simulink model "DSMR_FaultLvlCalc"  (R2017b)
settings: Solver=FixedStepDiscrete  StartTime=0.0  StopTime=10.0  FixedStep=0.02  RelTol=1e-3  EnableMultiTasking=on
undefined symbols (not defined in the file): bin2dec, BMS_DSMR_FaultLvlCalc, Delay, Delay1, DFES_Cls_DFC_638LinCommErr_C, DFES_Cls_DFC_AcDischgFobd_C, DFES_Cls_DFC_AChgFobd_C, DFES_Cls_DFC_AChgHVOffTmt_C, DFES_Cls_DFC_AChgHVOnTmt_C, DFES_Cls_DFC_AChgingErr_C, DFES_Cls_DFC_AChgLckTmt_C, DFES_Cls_DFC_AChgPileRdyTmt_C, DFES_Cls_DFC_AChgRdyPndiTmt_C, DFES_Cls_DFC_AChgRdyTmt_C, DFES_Cls_DFC_AChgS2ClsdTmt_C, DFES_Cls_DFC_AChgUnlckTmt_C, DFES_Cls_DFC_AChrgCnntErr_C, DFES_Cls_DFC_AChrgCurrMish_C, DFES_Cls_DFC_AChrgPortOvrTemp_C, DFES_Cls_DFC_AChrgVoltMish_C, DFES_Cls_DFC_AFEAdcRelatedErr_C, DFES_Cls_DFC_AFECellTempUpdErr_C, DFES_Cls_DFC_AFECellVoltLineOpen_C, DFES_Cls_DFC_AFECellVoltUpdErr_C, DFES_Cls_DFC_AFEComLost_C, DFES_Cls_DFC_AFEDiagModeExitErr_C, DFES_Cls_DFC_AFEGpioLineOpen_C, DFES_Cls_DFC_AFEOtherErr_C, DFES_Cls_DFC_AFEResetFlt_C, DFES_Cls_DFC_AFESampleErr_C, DFES_Cls_DFC_AFESplyFlt_C, DFES_Cls_DFC_AFETempHighFlt_C, DFES_Cls_DFC_APlusChk_C, DFES_Cls_DFC_BalCirOpenFlt_C, DFES_Cls_DFC_BalCirShortFlt_C, DFES_Cls_DFC_BalStuckMax_C, DFES_Cls_DFC_BalStuckMin_C, DFES_Cls_DFC_BalTempHighFlt_C, DFES_Cls_DFC_BattCurrMismatchErr_C, DFES_Cls_DFC_BattHVMsgTmt_C, DFES_Cls_DFC_BattSohChk_C, DFES_Cls_DFC_BattTAlrmMax_C, DFES_Cls_DFC_BattTAlrmMin_C, DFES_Cls_DFC_BattTCnstMax_C, DFES_Cls_DFC_BattTempVldMax_C, DFES_Cls_DFC_BattTempVldMin_C, DFES_Cls_DFC_BattTFaultMax_C, DFES_Cls_DFC_BattTFaultMin_C, DFES_Cls_DFC_BattTGradtMax_C, DFES_Cls_DFC_BattTHopMax_C, DFES_Cls_DFC_BattTWarnMax_C, DFES_Cls_DFC_BattTWarnMin_C, DFES_Cls_DFC_BattUNpl_C, DFES_Cls_DFC_BattVoltHiMax_C, DFES_Cls_DFC_BattVoltLoMin_C, DFES_Cls_DFC_BattVoltRngErr_C, DFES_Cls_DFC_BattVoltVld_C, DFES_Cls_DFC_BMSSplyPwrAbnToCAB_C, DFES_Cls_DFC_BMSSplyPwrAbnToLem_C, DFES_Cls_DFC_BoardTempTmt_C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
libraries: simulink x535
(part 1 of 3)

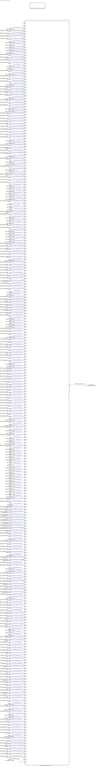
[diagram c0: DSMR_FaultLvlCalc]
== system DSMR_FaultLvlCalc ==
  DFC_CurrRngErr : Inport
  DFC_BattVoltRngErr : Inport  Port=2
  DFC_BattHVMsgTmt : Inport  Port=3
  DFC_BusHVMsgTmt : Inport  Port=4
  DFC_638LinCommErr : Inport  Port=5
  DFC_CellTempTmt : Inport  Port=6
  DFC_CellVoltTmt : Inport  Port=7
  DFC_InCanBusOff : Inport  Port=8
  DFC_VeCanBusOff : Inport  Port=9
  DFC_Msg2A3Tmt : Inport  Port=10
  DFC_RcMsg2A3Mis : Inport  Port=11
  DFC_ChkSumMsg2A3Err : Inport  Port=12
  DFC_RcMsg2A5Mis : Inport  Port=13
  DFC_RcMsg2A7Mis : Inport  Port=14
  DFC_CrashNpl : Inport  Port=15
  DFC_FuseNpl : Inport  Port=16
  DFC_Kl30cVoltLoErr : Inport  Port=17
  DFC_PosStuckMax : Inport  Port=18
  DFC_MPosStuckMin : Inport  Port=19
  DFC_MNegStuckMax : Inport  Port=20
  DFC_MNegStuckMin : Inport  Port=21
  DFC_PrStuckMin : Inport  Port=22
  DFC_DChrgPosStuckMax : Inport  Port=23
  DFC_DChrgPosStuckMin : Inport  Port=24
  DFC_DChrgNegStuckMax : Inport  Port=25
  DFC_DChrgNegStuckMin : Inport  Port=26
  DFC_HvPwrUpFail : Inport  Port=27
  DFC_DChrgPwrUpFail : Inport  Port=28
  DFC_BattTAlrmMax : Inport  Port=29
  DFC_BattTFaultMax : Inport  Port=30
  DFC_BattTAlrmMin : Inport  Port=31
  DFC_BattTFaultMin : Inport  Port=32
  DFC_BattTempVldMin : Inport  Port=33
  DFC_BattTCnstMax : Inport  Port=34
  DFC_BattTGradtMax : Inport  Port=35
  DFC_CellVoltAlrmMax : Inport  Port=36
  DFC_CellVoltFaultMax : Inport  Port=37
  DFC_CellVoltFusfMax : Inport  Port=38
  DFC_CellVoltAlrmMin : Inport  Port=39
  DFC_CellVoltFusfMin : Inport  Port=40
  DFC_CellVoltFaultMin : Inport  Port=41
  DFC_CellVoltVldMin : Inport  Port=42
  DFC_CellVoltNpl : Inport  Port=43
  DFC_Msg2E6Tmt : Inport  Port=44
  DFC_RcMsg2E6Mis : Inport  Port=45
  DFC_ChkSumMsg2E6Err : Inport  Port=46
  DFC_RcMsg2E1Mis : Inport  Port=47
  DFC_ChkSumMsg2E1Err : Inport  Port=48
  DFC_DcCanBusOff : Inport  Port=49
  DFC_DChrgTCnntMax : Inport  Port=50
  DFC_ChrgOCNpl : Inport  Port=51
  DFC_DisChOCNpl : Inport  Port=52
  DFC_BattVoltHiMax : Inport  Port=53
  DFC_BattVoltLoMin : Inport  Port=54
  DFC_ThmRnwy : Inport  Port=55
  DFC_AChrgPortOvrTemp : Inport  Port=56
  DFC_CurrOffsPlaus : Inport  Port=57
  DFC_CurrStukPlaus : Inport  Port=58
  DFC_CurrChrgPlaus : Inport  Port=59
  DFC_BattUNpl : Inport  Port=60
  DFC_BattVoltVld : Inport  Port=61
  DFC_PackUNpl : Inport  Port=62
  DFC_PackVoltVld : Inport  Port=63
  DFC_DChrgUNpl : Inport  Port=64
  DFC_DChrgVoltVld : Inport  Port=65
  DFC_BoardTempTmt : Inport  Port=66
  DFC_HvilMax : Inport  Port=67
  DFC_HvilMin : Inport  Port=68
  DFC_HvilSig : Inport  Port=69
  DFC_ChkSumMsg050Err : Inport  Port=70
  DFC_RcMsg050Mis : Inport  Port=71
  DFC_CrashHwNpl : Inport  Port=72
  DFC_IsoChkLv1 : Inport  Port=73
  DFC_IsoChkLv2 : Inport  Port=74
  DFC_InsResValdFault : Inport  Port=75
  DFC_Kl30OutRngErr : Inport  Port=76
  DFC_Kl30VoltLoErr : Inport  Port=77
  DFC_Kl30VoltHiErr : Inport  Port=78
  DFC_EepReadErr : Inport  Port=79
  DFC_BalStuckMax : Inport  Port=80
  DFC_BalStuckMin : Inport  Port=81
  DFC_CSCPwrSpyHiErr : Inport  Port=82
  DFC_CSCPwrSpyLoErr : Inport  Port=83
  DFC_CmcBordOTMax : Inport  Port=84
  DFC_BattTWarnMax : Inport  Port=85
  DFC_BattTWarnMin : Inport  Port=86
  DFC_BattTempVldMax : Inport  Port=87
  DFC_BattTHopMax : Inport  Port=88
  DFC_CellVoltRngHiErr : Inport  Port=89
  DFC_CellVoltRngLoErr : Inport  Port=90
  DFC_CellVoltWarnMax : Inport  Port=91
  DFC_CellVoltWarnMin : Inport  Port=92
  DFC_CellVoltVldMax : Inport  Port=93
  DFC_AChrgCurrMish : Inport  Port=94
  DFC_DChrgCurrMish : Inport  Port=95
  DFC_DChrgLowTempCurrMish : Inport  Port=96
  DFC_AChrgVoltMish : Inport  Port=97
  DFC_DChrgVoltMish : Inport  Port=98
  DFC_DChrgBattTMin : Inport  Port=99
  DFC_CC2Chk : Inport  Port=100
  DFC_APlusChk : Inport  Port=101
  DFC_DChrgMsgTmt : Inport  Port=102
  DFC_DChrgTNegElecMax : Inport  Port=103
  DFC_DChrgTNegElecMin : Inport  Port=104
  DFC_DChrgTNegElecSig : Inport  Port=105
  DFC_DChrgTPosElecMax : Inport  Port=106
  DFC_DChrgTPosElecMin : Inport  Port=107
  DFC_DChrgTPosElecSig : Inport  Port=108
  DFC_CcuSelfChkErr : Inport  Port=109
  DFC_ChrgOCMin : Inport  Port=110
  DFC_ChrgOCMax : Inport  Port=111
  DFC_DisChOCMin : Inport  Port=112
  DFC_DisChOCMax : Inport  Port=113
  DFC_SocRngLoMax : Inport  Port=114
  DFC_SocRngLoMin : Inport  Port=115
  DFC_SocRngHiMax : Inport  Port=116
  DFC_SocRngHiMin : Inport  Port=117
  DFC_InClntOverTmp : Inport  Port=118
  DFC_OutClntOverTmp : Inport  Port=119
  DFC_ClntDsTElecMax : Inport  Port=120
  DFC_ClntDsTElecMin : Inport  Port=121
  DFC_ClntDsTElecSig : Inport  Port=122
  DFC_ClntUsTElecMax : Inport  Port=123
  DFC_ClntUsTElecMin : Inport  Port=124
  DFC_ClntUsTElecSig : Inport  Port=125
  DFC_CoolPerfPlaus : Inport  Port=126
  DFC_HtgPerfPlaus : Inport  Port=127
  DFC_DChrgFobd : Inport  Port=128
  DFC_DChrgHvOnFail : Inport  Port=129
  DFC_AChgHVOnTmt : Inport  Port=130
  DFC_AChgHVOffTmt : Inport  Port=131
  DFC_AChgS2ClsdTmt : Inport  Port=132
  DFC_DChrgStakeErr : Inport  Port=133
  DFC_DChrgStkVoltErr : Inport  Port=134
  DFC_DChrgStkCurrErr : Inport  Port=135
  DFC_AChgPileRdyTmt : Inport  Port=136
  DFC_DChrgCHMTmt : Inport  Port=137
  DFC_DChrgCRMTmt : Inport  Port=138
  DFC_DChrgCMLTmt : Inport  Port=139
  DFC_DChrgCROTmt : Inport  Port=140
  DFC_DChrgCCSTmt : Inport  Port=141
  DFC_DChrgCSTTmt : Inport  Port=142
  DFC_DChrgCSDTmt : Inport  Port=143
  DFC_DChrgParaChk : Inport  Port=144
  DFC_DChrgCableChk : Inport  Port=145
  DFC_DChrgSLACTOut : Inport  Port=146
  DFC_DChrgCnntErr : Inport  Port=147
  DFC_DChrgLckErr : Inport  Port=148
  DFC_AChrgCnntErr : Inport  Port=149
  DFC_AChgLckTmt : Inport  Port=150
  DFC_AChgRdyPndiTmt : Inport  Port=151
  DFC_AChgRdyTmt : Inport  Port=152
  DFC_AChgingErr : Inport  Port=153
  DFC_AChgUnlckTmt : Inport  Port=154
  DFC_AChgFobd : Inport  Port=155
  DFC_SocValJmp : Inport  Port=156
  DFC_ChrgCmuLost : Inport  Port=157
  DFC_DisChrgCmuLost : Inport  Port=158
  DFC_Msg130Tmt : Inport  Port=159
  DFC_Msg2E1Tmt : Inport  Port=160
  DFC_Msg2EBTmt : Inport  Port=161
  DFC_MsgCABTmt : Inport  Port=162
  DFC_Msg0B5Tmt : Inport  Port=163
  DFC_ObcTmt : Inport  Port=164
  DFC_VcuTmt : Inport  Port=165
  DFC_Msg2A7Tmt : Inport  Port=166
  DFC_Msg2A5Tmt : Inport  Port=167
  DFC_Msg2ADTmt : Inport  Port=168
  DFC_Msg2BBTmt : Inport  Port=169
  DFC_Msg2DFTmt : Inport  Port=170
  DFC_Msg3AATmt : Inport  Port=171
  DFC_Msg050Tmt : Inport  Port=172
  DFC_Msg2F1Tmt : Inport  Port=173
  DFC_Msg195Tmt : Inport  Port=174
  DFC_Msg37FTmt : Inport  Port=175
  DFC_Msg28CTmt : Inport  Port=176
  DFC_Msg17DTmt : Inport  Port=177
  DFC_HwCurrElecSCG : Inport  Port=178
  DFC_HwCurrElecSCP : Inport  Port=179
  DFC_CABErr : Inport  Port=180
  DFC_BattCurrMismatchErr : Inport  Port=181
  GaCFM_AFEComLost_flg : Inport  Port=182
  GaCFM_AFECellVoltUpdErr_flg : Inport  Port=183
  GaCFM_AFECellTempUpdErr_flg : Inport  Port=184
  GaCFM_AFESampleErr_flg : Inport  Port=185
  GaCFM_AFECellVoltLineOpen_flg : Inport  Port=186
  GaCFM_AFEGpioLineOpen_flg : Inport  Port=187
  GaCFM_AFEAdcRelatedErr_flg : Inport  Port=188
  GaCFM_AFEDiagModeExitErr_flg : Inport  Port=189
  GaCFM_AFEOtherErr_flg : Inport  Port=190
  DFC_AcDischgFobd : Inport  Port=191
  DFC_BalCirOpenFlt : Inport  Port=192
  DFC_BalCirShortFlt : Inport  Port=193
  DFC_BalTempHighFlt : Inport  Port=194
  DFC_HVSmplComFlt : Inport  Port=195
  DFC_HVSmplSigErr : Inport  Port=196
  DFC_HVSmplSplyFlt : Inport  Port=197
  DFC_CABVoltOutOfRng : Inport  Port=198
  DFC_CABDevFlt : Inport  Port=199
  DFC_BMSSplyPwrAbnToLem : Inport  Port=200
  DFC_BMSSplyPwrAbnToCAB : Inport  Port=201
  DFC_NVMReadError : Inport  Port=202
  DFC_KL30Shutdown : Inport  Port=203
  DFC_MCUResetFlt : Inport  Port=204
  DFC_BattSohChk : Inport  Port=205
  DFC_CalCANBusOff : Inport  Port=206
  DFC_ThmRnwyWarn : Inport  Port=207
  DFC_PchgOvrCurrFlt : Inport  Port=208
  DFC_SBCSplyPwrOvrVolt : Inport  Port=209
  DFC_SBCSplyPwrUnderVolt : Inport  Port=210
  DFC_SBCSplyPwrOvrCurr : Inport  Port=211
  DFC_CrashChkHwFrqAbnorm : Inport  Port=212
  DFC_CrashChkHwDutyAbnorm : Inport  Port=213
  DFC_AFETempHighFlt : Inport  Port=214
  DFC_EVCCDevFlt : Inport  Port=215
  DFC_EVCCSplyPwrFlt : Inport  Port=216
  DFC_EVCCVehComFlt : Inport  Port=217
  DFC_EVCCPileComFlt : Inport  Port=218
  DFC_EVCCVehHwFlt : Inport  Port=219
  DFC_EVCCPileHwFlt : Inport  Port=220
  DFC_IsoS1SwStuckOpen : Inport  Port=221
  DFC_IsoS1SwStuckClsd : Inport  Port=222
  DFC_IsoS2SwStuckOpen : Inport  Port=223
  DFC_IsoS2SwStuckClsd : Inport  Port=224
  DFC_IsoS3SwStuckOpen : Inport  Port=225
  DFC_IsoS3SwStuckClsd : Inport  Port=226
  DFC_AFEResetFlt : Inport  Port=227
  DFC_AFESplyFlt : Inport  Port=228
  DFC_PreHeatErr : Inport  Port=229
  DFC_PreHeatVcuReqTmt : Inport  Port=230
  DFC_PreHeatObcStatusErr : Inport  Port=231
  DFC_PreHeatPtcErr : Inport  Port=232
  DFC_MPosRlyDrvScb : Inport  Port=233
  DFC_MPosRlyDrvScg : Inport  Port=234
  DFC_MPosRlyDrvOL : Inport  Port=235
  DFC_MposRlyDrvOvrCurr : Inport  Port=236
  DFC_MPosRlyDrvFault : Inport  Port=237
  DFC_MNegRlyDrvScb : Inport  Port=238
  DFC_MNegRlyDrvScg : Inport  Port=239
  DFC_MNegRlyDrvOL : Inport  Port=240
  DFC_MNegRlyDrvOvrCurr : Inport  Port=241
  DFC_MNegRlyDrvFault : Inport  Port=242
  DFC_DcPosRlyDrvScb : Inport  Port=243
  DFC_DcPosRlyDrvScg : Inport  Port=244
  DFC_DcPosRlyDrvOL : Inport  Port=245
  DFC_DChrgPosRlyDrvOvrCurr : Inport  Port=246
  DFC_DcPosRlyDrvFault : Inport  Port=247
  DFC_DcNegRlyDrvScb : Inport  Port=248
  DFC_DcNegRlyDrvScg : Inport  Port=249
  DFC_DcNegRlyDrvOL : Inport  Port=250
  DFC_DChrgNegRlyDrvOvrCurr : Inport  Port=251
  DFC_DcNegRlyDrvFault : Inport  Port=252
  DFC_PreRlyDrvScb : Inport  Port=253
  DFC_PreRlyDrvScg : Inport  Port=254
  DFC_PreRlyDrvOL : Inport  Port=255
  DFC_PrRlyDrvOvrCurr : Inport  Port=256
  DFC_CellTAlrmMax : Inport  Port=257
  DFC_CellTFaultMax : Inport  Port=258
  DFC_CellTAlrmMin : Inport  Port=259
  DFC_CellTFaultMin : Inport  Port=260
  DFC_CellTempVldMin : Inport  Port=261
  DFC_CellTCnstMax : Inport  Port=262
  DFC_CellTGradtMax : Inport  Port=263
  DFC_CellTWarnMax : Inport  Port=264
  DFC_CellTWarnMin : Inport  Port=265
  DFC_CellTempVldMax : Inport  Port=266
  DFC_CellTHopMax : Inport  Port=267
  DFC_TwoCurrSnsrFlt : Inport  Port=268
  DFC_ThmRnwyAlarm : Inport  Port=269
  DFC_ChkSumMsg2A5Err : Inport  Port=270
  DFC_ChkSumMsg2A7Err : Inport  Port=271
  DFC_DchrgIsoChkLv1 : Inport  Port=272
  DFC_DchrgIsoChkLv2 : Inport  Port=273
  DFC_HVOffIsoChkLv1 : Inport  Port=274
  DFC_HVOffIsoChkLv2 : Inport  Port=275
  DFC_PackCrntSaf : Inport  Port=276
  BMS_DSMR_FaultLvlCalc : Subsystem
  FaultLvlCoord_Clear_Function : Subsystem  TreatAsAtomicUnit=on
  DSMR_stFaultRank : Outport
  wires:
  DFC_CurrRngErr/1 -> BMS_DSMR_FaultLvlCalc/1(DFC_CurrRngErr)  "DFC_CurrRngErr"
  DFC_BattVoltRngErr/1 -> BMS_DSMR_FaultLvlCalc/2(DFC_BattVoltRngErr)  "DFC_BattVoltRngErr"
  DFC_BattHVMsgTmt/1 -> BMS_DSMR_FaultLvlCalc/3(DFC_BattHVMsgTmt)  "DFC_BattHVMsgTmt"
  DFC_BusHVMsgTmt/1 -> BMS_DSMR_FaultLvlCalc/4(DFC_BusHVMsgTmt)  "DFC_BusHVMsgTmt"
  DFC_638LinCommErr/1 -> BMS_DSMR_FaultLvlCalc/5(DFC_638LinCommErr)  "DFC_638LinCommErr"
  DFC_CellTempTmt/1 -> BMS_DSMR_FaultLvlCalc/6(DFC_CellTempTmt)  "DFC_CellTempTmt"
  DFC_CellVoltTmt/1 -> BMS_DSMR_FaultLvlCalc/7(DFC_CellVoltTmt)  "DFC_CellVoltTmt"
  DFC_InCanBusOff/1 -> BMS_DSMR_FaultLvlCalc/8(DFC_InCanBusOff)  "DFC_InCanBusOff"
  DFC_VeCanBusOff/1 -> BMS_DSMR_FaultLvlCalc/9(DFC_VeCanBusOff)  "DFC_VeCanBusOff"
  DFC_Msg2A3Tmt/1 -> BMS_DSMR_FaultLvlCalc/10(DFC_Msg2A3Tmt)  "DFC_Msg2A3Tmt"
  DFC_RcMsg2A3Mis/1 -> BMS_DSMR_FaultLvlCalc/11(DFC_RcMsg2A3Mis)  "DFC_RcMsg2A3Mis"
  DFC_ChkSumMsg2A3Err/1 -> BMS_DSMR_FaultLvlCalc/12(DFC_ChkSumMsg2A3Err)  "DFC_ChkSumMsg2A3Err"
  DFC_RcMsg2A5Mis/1 -> BMS_DSMR_FaultLvlCalc/13(DFC_RcMsg2A5Mis)  "DFC_RcMsg2A5Mis"
  DFC_RcMsg2A7Mis/1 -> BMS_DSMR_FaultLvlCalc/14(DFC_RcMsg2A7Mis)  "DFC_RcMsg2A7Mis"
  DFC_CrashNpl/1 -> BMS_DSMR_FaultLvlCalc/15(DFC_CrashNpl)  "DFC_CrashNpl"
  DFC_FuseNpl/1 -> BMS_DSMR_FaultLvlCalc/16(DFC_FuseNpl)  "DFC_FuseNpl"
  DFC_Kl30cVoltLoErr/1 -> BMS_DSMR_FaultLvlCalc/17(DFC_Kl30cVoltLoErr)  "DFC_Kl30cVoltLoErr"
  DFC_PosStuckMax/1 -> BMS_DSMR_FaultLvlCalc/18(DFC_PosStuckMax)  "DFC_PosStuckMax"
  DFC_MPosStuckMin/1 -> BMS_DSMR_FaultLvlCalc/19(DFC_MPosStuckMin)  "DFC_MPosStuckMin"
  DFC_MNegStuckMax/1 -> BMS_DSMR_FaultLvlCalc/20(DFC_MNegStuckMax)  "DFC_MNegStuckMax"
  DFC_MNegStuckMin/1 -> BMS_DSMR_FaultLvlCalc/21(DFC_MNegStuckMin)  "DFC_MNegStuckMin"
  DFC_PrStuckMin/1 -> BMS_DSMR_FaultLvlCalc/22(DFC_PrStuckMin)  "DFC_PrStuckMin"
  DFC_DChrgPosStuckMax/1 -> BMS_DSMR_FaultLvlCalc/23(DFC_DChrgPosStuckMax)  "DFC_DChrgPosStuckMax"
  DFC_DChrgPosStuckMin/1 -> BMS_DSMR_FaultLvlCalc/24(DFC_DChrgPosStuckMin)  "DFC_DChrgPosStuckMin"
  DFC_DChrgNegStuckMax/1 -> BMS_DSMR_FaultLvlCalc/25(DFC_DChrgNegStuckMax)  "DFC_DChrgNegStuckMax"
  DFC_DChrgNegStuckMin/1 -> BMS_DSMR_FaultLvlCalc/26(DFC_DChrgNegStuckMin)  "DFC_DChrgNegStuckMin"
  DFC_HvPwrUpFail/1 -> BMS_DSMR_FaultLvlCalc/27(DFC_HvPwrUpFail)  "DFC_HvPwrUpFail"
  DFC_DChrgPwrUpFail/1 -> BMS_DSMR_FaultLvlCalc/28(DFC_DChrgPwrUpFail)  "DFC_DChrgPwrUpFail"
  DFC_BattTAlrmMax/1 -> BMS_DSMR_FaultLvlCalc/29(DFC_BattTAlrmMax)  "DFC_BattTAlrmMax"
  DFC_BattTFaultMax/1 -> BMS_DSMR_FaultLvlCalc/30(DFC_BattTFaultMax)  "DFC_BattTFaultMax"
  DFC_BattTAlrmMin/1 -> BMS_DSMR_FaultLvlCalc/31(DFC_BattTAlrmMin)  "DFC_BattTAlrmMin"
  DFC_BattTFaultMin/1 -> BMS_DSMR_FaultLvlCalc/32(DFC_BattTFaultMin)  "DFC_BattTFaultMin"
  DFC_BattTempVldMin/1 -> BMS_DSMR_FaultLvlCalc/33(DFC_BattTempVldMin)  "DFC_BattTempVldMin"
  DFC_BattTCnstMax/1 -> BMS_DSMR_FaultLvlCalc/34(DFC_BattTCnstMax)  "DFC_BattTCnstMax"
  DFC_BattTGradtMax/1 -> BMS_DSMR_FaultLvlCalc/35(DFC_BattTGradtMax)  "DFC_BattTGradtMax"
  DFC_CellVoltAlrmMax/1 -> BMS_DSMR_FaultLvlCalc/36(DFC_CellVoltAlrmMax)  "DFC_CellVoltAlrmMax"
  DFC_CellVoltFaultMax/1 -> BMS_DSMR_FaultLvlCalc/37(DFC_CellVoltFaultMax)  "DFC_CellVoltFaultMax"
  DFC_CellVoltFusfMax/1 -> BMS_DSMR_FaultLvlCalc/38(DFC_CellVoltFusfMax)  "DFC_CellVoltFusfMax"
  DFC_CellVoltAlrmMin/1 -> BMS_DSMR_FaultLvlCalc/39(DFC_CellVoltAlrmMin)  "DFC_CellVoltAlrmMin"
  DFC_CellVoltFusfMin/1 -> BMS_DSMR_FaultLvlCalc/40(DFC_CellVoltFusfMin)  "DFC_CellVoltFusfMin"
  DFC_CellVoltFaultMin/1 -> BMS_DSMR_FaultLvlCalc/41(DFC_CellVoltFaultMin)  "DFC_CellVoltFaultMin"
  DFC_CellVoltVldMin/1 -> BMS_DSMR_FaultLvlCalc/42(DFC_CellVoltVldMin)  "DFC_CellVoltVldMin"
  DFC_CellVoltNpl/1 -> BMS_DSMR_FaultLvlCalc/43(DFC_CellVoltNpl)  "DFC_CellVoltNpl"
  DFC_Msg2E6Tmt/1 -> BMS_DSMR_FaultLvlCalc/44(DFC_Msg2E6Tmt)  "DFC_Msg2E6Tmt"
  DFC_RcMsg2E6Mis/1 -> BMS_DSMR_FaultLvlCalc/45(DFC_RcMsg2E6Mis)  "DFC_RcMsg2E0Mis"
  DFC_ChkSumMsg2E6Err/1 -> BMS_DSMR_FaultLvlCalc/46(DFC_ChkSumMsg2E6Err)  "DFC_ChkSumMsg2E0Err"
  DFC_RcMsg2E1Mis/1 -> BMS_DSMR_FaultLvlCalc/47(DFC_RcMsg2E1Mis)  "DFC_RcMsg2E1Mis"
  DFC_ChkSumMsg2E1Err/1 -> BMS_DSMR_FaultLvlCalc/48(DFC_ChkSumMsg2E1Err)  "DFC_ChkSumMsg2E1Err"
  DFC_DcCanBusOff/1 -> BMS_DSMR_FaultLvlCalc/49(DFC_DcCanBusOff)  "DFC_DcCanBusOff"
  DFC_DChrgTCnntMax/1 -> BMS_DSMR_FaultLvlCalc/50(DFC_DChrgTCnntMax)  "DFC_DChrgTCnntMax"
  DFC_ChrgOCNpl/1 -> BMS_DSMR_FaultLvlCalc/51(DFC_ChrgOCNpl)  "DFC_ChrgOCNpl"
  DFC_DisChOCNpl/1 -> BMS_DSMR_FaultLvlCalc/52(DFC_DisChOCNpl)  "DFC_DisChOCNpl"
  DFC_BattVoltHiMax/1 -> BMS_DSMR_FaultLvlCalc/53(DFC_BattVoltHiMax)  "DFC_BattVoltHiMax"
  DFC_BattVoltLoMin/1 -> BMS_DSMR_FaultLvlCalc/54(DFC_BattVoltLoMin)  "DFC_BattVoltLoMin"
  DFC_ThmRnwy/1 -> BMS_DSMR_FaultLvlCalc/55(DFC_ThmRnwy)  "DFC_ThmRnwy"
  DFC_AChrgPortOvrTemp/1 -> BMS_DSMR_FaultLvlCalc/56(DFC_AChrgPortOvrTemp)  "DFC_AChrgPortOvrTemp"
  DFC_CurrOffsPlaus/1 -> BMS_DSMR_FaultLvlCalc/57(DFC_CurrOffsPlaus)  "DFC_CurrOffsPlaus"
  DFC_CurrStukPlaus/1 -> BMS_DSMR_FaultLvlCalc/58(DFC_CurrStukPlaus)  "DFC_CurrStukPlaus"
  DFC_CurrChrgPlaus/1 -> BMS_DSMR_FaultLvlCalc/59(DFC_CurrChrgPlaus)  "DFC_CurrChrgPlaus"
  DFC_BattUNpl/1 -> BMS_DSMR_FaultLvlCalc/60(DFC_BattUNpl)  "DFC_BattUNpl"
  DFC_BattVoltVld/1 -> BMS_DSMR_FaultLvlCalc/61(DFC_BattVoltVld)  "DFC_BattVoltVld"
  DFC_PackUNpl/1 -> BMS_DSMR_FaultLvlCalc/62(DFC_PackUNpl)  "DFC_PackUNpl"
  DFC_PackVoltVld/1 -> BMS_DSMR_FaultLvlCalc/63(DFC_PackVoltVld)  "DFC_PackVoltVld"
  DFC_DChrgUNpl/1 -> BMS_DSMR_FaultLvlCalc/64(DFC_DChrgUNpl)  "DFC_DChrgUNpl"
  DFC_DChrgVoltVld/1 -> BMS_DSMR_FaultLvlCalc/65(DFC_DChrgVoltVld)  "DFC_DChrgVoltVld"
  DFC_BoardTempTmt/1 -> BMS_DSMR_FaultLvlCalc/66(DFC_BoardTempTmt)  "DFC_BoardTempTmt"
  DFC_HvilMax/1 -> BMS_DSMR_FaultLvlCalc/67(DFC_HvilMax)  "DFC_HvilMax"
  DFC_HvilMin/1 -> BMS_DSMR_FaultLvlCalc/68(DFC_HvilMin)  "DFC_HvilMin"
  DFC_HvilSig/1 -> BMS_DSMR_FaultLvlCalc/69(DFC_HvilSig)  "DFC_HvilSig"
  DFC_ChkSumMsg050Err/1 -> BMS_DSMR_FaultLvlCalc/70(DFC_ChkSumMsg050Err)  "DFC_ChkSumMsg050Err"
  DFC_RcMsg050Mis/1 -> BMS_DSMR_FaultLvlCalc/71(DFC_RcMsg050Mis)  "DFC_RcMsg050Mis"
  DFC_CrashHwNpl/1 -> BMS_DSMR_FaultLvlCalc/72(DFC_CrashHwNpl)  "DFC_CrashHwNpl"
  DFC_IsoChkLv1/1 -> BMS_DSMR_FaultLvlCalc/73(DFC_IsoChkLv1)  "DFC_IsoChkLv1"
  DFC_IsoChkLv2/1 -> BMS_DSMR_FaultLvlCalc/74(DFC_IsoChkLv2)  "DFC_IsoChkLv2"
  DFC_InsResValdFault/1 -> BMS_DSMR_FaultLvlCalc/75(DFC_InsResValdFault)  "DFC_InsResValdFault"
  DFC_Kl30OutRngErr/1 -> BMS_DSMR_FaultLvlCalc/76(DFC_Kl30OutRngErr)  "DFC_Kl30OutRngErr"
  DFC_Kl30VoltLoErr/1 -> BMS_DSMR_FaultLvlCalc/77(DFC_Kl30VoltLoErr)  "DFC_Kl30VoltLoErr"
  DFC_Kl30VoltHiErr/1 -> BMS_DSMR_FaultLvlCalc/78(DFC_Kl30VoltHiErr)  "DFC_Kl30VoltHiErr"
  DFC_EepReadErr/1 -> BMS_DSMR_FaultLvlCalc/79(DFC_EepReadErr)  "DFC_EepReadErr"
  DFC_BalStuckMax/1 -> BMS_DSMR_FaultLvlCalc/80(DFC_BalStuckMax)  "DFC_BalStuckMax"
  DFC_BalStuckMin/1 -> BMS_DSMR_FaultLvlCalc/81(DFC_BalStuckMin)  "DFC_BalStuckMin"
  DFC_CSCPwrSpyHiErr/1 -> BMS_DSMR_FaultLvlCalc/82(DFC_CSCPwrSpyHiErr)  "DFC_CSCPwrSpyHiErr"
  DFC_CSCPwrSpyLoErr/1 -> BMS_DSMR_FaultLvlCalc/83(DFC_CSCPwrSpyLoErr)  "DFC_CSCPwrSpyLoErr"
  DFC_CmcBordOTMax/1 -> BMS_DSMR_FaultLvlCalc/84(DFC_CmcBordOTMax)  "DFC_CmcBordOTMax"
  DFC_BattTWarnMax/1 -> BMS_DSMR_FaultLvlCalc/85(DFC_BattTWarnMax)  "DFC_BattTWarnMax"
  DFC_BattTWarnMin/1 -> BMS_DSMR_FaultLvlCalc/86(DFC_BattTWarnMin)  "DFC_BattTWarnMin"
  DFC_BattTempVldMax/1 -> BMS_DSMR_FaultLvlCalc/87(DFC_BattTempVldMax)  "DFC_BattTempVldMax"
  DFC_BattTHopMax/1 -> BMS_DSMR_FaultLvlCalc/88(DFC_BattTHopMax)  "DFC_BattTHopMax"
  DFC_CellVoltRngHiErr/1 -> BMS_DSMR_FaultLvlCalc/89(DFC_CellVoltRngHiErr)  "DFC_CellVoltRngHiErr"
  DFC_CellVoltRngLoErr/1 -> BMS_DSMR_FaultLvlCalc/90(DFC_CellVoltRngLoErr)  "DFC_CellVoltRngLoErr"
  DFC_CellVoltWarnMax/1 -> BMS_DSMR_FaultLvlCalc/91(DFC_CellVoltWarnMax)  "DFC_CellVoltWarnMax"
  DFC_CellVoltWarnMin/1 -> BMS_DSMR_FaultLvlCalc/92(DFC_CellVoltWarnMin)  "DFC_CellVoltWarnMin"
  DFC_CellVoltVldMax/1 -> BMS_DSMR_FaultLvlCalc/93(DFC_CellVoltVldMax)  "DFC_CellVoltVldMax"
  DFC_AChrgCurrMish/1 -> BMS_DSMR_FaultLvlCalc/94(DFC_AChrgCurrMish)  "DFC_AChrgCurrMish"
  DFC_DChrgCurrMish/1 -> BMS_DSMR_FaultLvlCalc/95(DFC_DChrgCurrMish)  "DFC_DChrgCurrMish"
  DFC_DChrgLowTempCurrMish/1 -> BMS_DSMR_FaultLvlCalc/96(DFC_DChrgLowTempCurrMish)  "DFC_DChrgLowTempCurrMish"
  DFC_AChrgVoltMish/1 -> BMS_DSMR_FaultLvlCalc/97(DFC_AChrgVoltMish)  "DFC_AChrgVoltMish"
  DFC_DChrgVoltMish/1 -> BMS_DSMR_FaultLvlCalc/98(DFC_DChrgVoltMish)  "DFC_DChrgVoltMish"
  DFC_DChrgBattTMin/1 -> BMS_DSMR_FaultLvlCalc/99(DFC_DChrgBattTMin)  "DFC_DChrgBattTMin"
  DFC_CC2Chk/1 -> BMS_DSMR_FaultLvlCalc/100(DFC_CC2Chk)  "DFC_CC2Chk"
  DFC_APlusChk/1 -> BMS_DSMR_FaultLvlCalc/101(DFC_APlusChk)  "DFC_APlusChk"
  DFC_DChrgMsgTmt/1 -> BMS_DSMR_FaultLvlCalc/102(DFC_DChrgMsgTmt)  "DFC_DChrgMsgTmt"
  DFC_DChrgTNegElecMax/1 -> BMS_DSMR_FaultLvlCalc/103(DFC_DChrgTNegElecMax)  "DFC_DChrgTNegElecMax"
  DFC_DChrgTNegElecMin/1 -> BMS_DSMR_FaultLvlCalc/104(DFC_DChrgTNegElecMin)  "DFC_DChrgTNegElecMin"
  DFC_DChrgTNegElecSig/1 -> BMS_DSMR_FaultLvlCalc/105(DFC_DChrgTNegElecSig)  "DFC_DChrgTNegElecSig"
  DFC_DChrgTPosElecMax/1 -> BMS_DSMR_FaultLvlCalc/106(DFC_DChrgTPosElecMax)  "DFC_DChrgTPosElecMax"
  DFC_DChrgTPosElecMin/1 -> BMS_DSMR_FaultLvlCalc/107(DFC_DChrgTPosElecMin)  "DFC_DChrgTPosElecMin"
  DFC_DChrgTPosElecSig/1 -> BMS_DSMR_FaultLvlCalc/108(DFC_DChrgTPosElecSig)  "DFC_DChrgTPosElecSig"
  DFC_CcuSelfChkErr/1 -> BMS_DSMR_FaultLvlCalc/109(DFC_CcuSelfChkErr)  "DFC_CcuSelfChkErr"
  DFC_ChrgOCMin/1 -> BMS_DSMR_FaultLvlCalc/110(DFC_ChrgOCMin)  "DFC_ChrgOCMin"
  DFC_ChrgOCMax/1 -> BMS_DSMR_FaultLvlCalc/111(DFC_ChrgOCMax)  "DFC_ChrgOCMax"
  DFC_DisChOCMin/1 -> BMS_DSMR_FaultLvlCalc/112(DFC_DisChOCMin)  "DFC_DisChOCMin"
  DFC_DisChOCMax/1 -> BMS_DSMR_FaultLvlCalc/113(DFC_DisChOCMax)  "DFC_DisChOCMax"
  DFC_SocRngLoMax/1 -> BMS_DSMR_FaultLvlCalc/114(DFC_SocRngLoMax)  "DFC_SocRngLoMax"
  DFC_SocRngLoMin/1 -> BMS_DSMR_FaultLvlCalc/115(DFC_SocRngLoMin)  "DFC_SocRngLoMin"
  DFC_SocRngHiMax/1 -> BMS_DSMR_FaultLvlCalc/116(DFC_SocRngHiMax)  "DFC_SocRngHiMax"
  DFC_SocRngHiMin/1 -> BMS_DSMR_FaultLvlCalc/117(DFC_SocRngHiMin)  "DFC_SocRngHiMin"
  DFC_InClntOverTmp/1 -> BMS_DSMR_FaultLvlCalc/118(DFC_InClntOverTmp)  "DFC_InClntOverTmp"
  DFC_OutClntOverTmp/1 -> BMS_DSMR_FaultLvlCalc/119(DFC_OutClntOverTmp)  "DFC_OutClntOverTmp"
  DFC_ClntDsTElecMax/1 -> BMS_DSMR_FaultLvlCalc/120(DFC_ClntDsTElecMax)  "DFC_ClntDsTElecMax"
  DFC_ClntDsTElecMin/1 -> BMS_DSMR_FaultLvlCalc/121(DFC_ClntDsTElecMin)  "DFC_ClntDsTElecMin"
  DFC_ClntDsTElecSig/1 -> BMS_DSMR_FaultLvlCalc/122(DFC_ClntDsTElecSig)  "DFC_ClntDsTElecSig"
  DFC_ClntUsTElecMax/1 -> BMS_DSMR_FaultLvlCalc/123(DFC_ClntUsTElecMax)  "DFC_ClntUsTElecMax"
  DFC_ClntUsTElecMin/1 -> BMS_DSMR_FaultLvlCalc/124(DFC_ClntUsTElecMin)  "DFC_ClntUsTElecMin"
  DFC_ClntUsTElecSig/1 -> BMS_DSMR_FaultLvlCalc/125(DFC_ClntUsTElecSig)  "DFC_ClntUsTElecSig"
  DFC_CoolPerfPlaus/1 -> BMS_DSMR_FaultLvlCalc/126(DFC_CoolPerfPlaus)  "DFC_CoolPerfPlaus"
  DFC_HtgPerfPlaus/1 -> BMS_DSMR_FaultLvlCalc/127(DFC_HtgPerfPlaus)  "DFC_HtgPerfPlaus"
  DFC_DChrgFobd/1 -> BMS_DSMR_FaultLvlCalc/128(DFC_DChrgFobd)  "DFC_DChrgFobd"
  DFC_DChrgHvOnFail/1 -> BMS_DSMR_FaultLvlCalc/129(DFC_DChrgHvOnFail)  "DFC_DChrgHvOnFail"
  DFC_AChgHVOnTmt/1 -> BMS_DSMR_FaultLvlCalc/130(DFC_AChgHVOnTmt)  "DFC_AChgHVOnTmt"
  DFC_AChgHVOffTmt/1 -> BMS_DSMR_FaultLvlCalc/131(DFC_AChgHVOffTmt)  "DFC_AChgHVOffTmt"
  DFC_AChgS2ClsdTmt/1 -> BMS_DSMR_FaultLvlCalc/132(DFC_AChgS2ClsdTmt)  "DFC_AChgS2ClsdTmt"
  DFC_DChrgStakeErr/1 -> BMS_DSMR_FaultLvlCalc/133(DFC_DChrgStakeErr)  "DFC_DChrgStakeErr"
  DFC_DChrgStkVoltErr/1 -> BMS_DSMR_FaultLvlCalc/134(DFC_DChrgStkVoltErr)  "DFC_DChrgStkVoltErr"
  DFC_DChrgStkCurrErr/1 -> BMS_DSMR_FaultLvlCalc/135(DFC_DChrgStkCurrErr)  "DFC_DChrgStkCurrErr"
  DFC_AChgPileRdyTmt/1 -> BMS_DSMR_FaultLvlCalc/136(DFC_AChgPileRdyTmt)  "DFC_AChgPileRdyTmt"
  DFC_DChrgCHMTmt/1 -> BMS_DSMR_FaultLvlCalc/137(DFC_DChrgCHMTmt)  "DFC_DChrgCHMTmt"
  DFC_DChrgCRMTmt/1 -> BMS_DSMR_FaultLvlCalc/138(DFC_DChrgCRMTmt)  "DFC_DChrgCRMTmt"
  DFC_DChrgCMLTmt/1 -> BMS_DSMR_FaultLvlCalc/139(DFC_DChrgCMLTmt)  "DFC_DChrgCMLTmt"
  DFC_DChrgCROTmt/1 -> BMS_DSMR_FaultLvlCalc/140(DFC_DChrgCROTmt)  "DFC_DChrgCROTmt"
  DFC_DChrgCCSTmt/1 -> BMS_DSMR_FaultLvlCalc/141(DFC_DChrgCCSTmt)  "DFC_DChrgCCSTmt"
  DFC_DChrgCSTTmt/1 -> BMS_DSMR_FaultLvlCalc/142(DFC_DChrgCSTTmt)  "DFC_DChrgCSTTmt"
  DFC_DChrgCSDTmt/1 -> BMS_DSMR_FaultLvlCalc/143(DFC_DChrgCSDTmt)  "DFC_DChrgCSDTmt"
  DFC_DChrgParaChk/1 -> BMS_DSMR_FaultLvlCalc/144(DFC_DChrgParaChk)  "DFC_DChrgParaChk"
  DFC_DChrgCableChk/1 -> BMS_DSMR_FaultLvlCalc/145(DFC_DChrgCableChk)  "DFC_DChrgCableChk"
  DFC_DChrgSLACTOut/1 -> BMS_DSMR_FaultLvlCalc/146(DFC_DChrgSLACTOut)  "DFC_DChrgSLACTOut"
  DFC_DChrgCnntErr/1 -> BMS_DSMR_FaultLvlCalc/147(DFC_DChrgCnntErr)  "DFC_DChrgCnntErr"
  DFC_DChrgLckErr/1 -> BMS_DSMR_FaultLvlCalc/148(DFC_DChrgLckErr)  "DFC_DChrgLckErr"
  DFC_AChrgCnntErr/1 -> BMS_DSMR_FaultLvlCalc/149(DFC_AChrgCnntErr)  "DFC_AChrgCnntErr"
  DFC_AChgLckTmt/1 -> BMS_DSMR_FaultLvlCalc/150(DFC_AChgLckTmt)  "DFC_AChgLckTmt"
  DFC_AChgRdyPndiTmt/1 -> BMS_DSMR_FaultLvlCalc/151(DFC_AChgRdyPndiTmt)  "DFC_AChgRdyPndiTmt"
  DFC_AChgRdyTmt/1 -> BMS_DSMR_FaultLvlCalc/152(DFC_AChgRdyTmt)  "DFC_AChgRdyTmt"
  DFC_AChgingErr/1 -> BMS_DSMR_FaultLvlCalc/153(DFC_AChgingErr)  "DFC_AChgingErr"
  DFC_AChgUnlckTmt/1 -> BMS_DSMR_FaultLvlCalc/154(DFC_AChgUnlckTmt)  "DFC_AChgUnlckTmt"
  DFC_AChgFobd/1 -> BMS_DSMR_FaultLvlCalc/155(DFC_AChgFobd)  "DFC_AChgFobd"
  DFC_SocValJmp/1 -> BMS_DSMR_FaultLvlCalc/156(DFC_SocValJmp)  "DFC_SocValJmp"
  BMS_DSMR_FaultLvlCalc/1(DSMR_stFaultRank) -> DSMR_stFaultRank/1  "DSMR_stFaultRank"
  DFC_ChrgCmuLost/1 -> BMS_DSMR_FaultLvlCalc/157(DFC_ChrgCmuLost)  "DFC_ChrgCmuLost"
  DFC_DisChrgCmuLost/1 -> BMS_DSMR_FaultLvlCalc/158(DFC_DisChrgCmuLost)  "DFC_DisChrgCmuLost"
  DFC_MsgCABTmt/1 -> BMS_DSMR_FaultLvlCalc/162(DFC_MsgCABTmt)  "DFC_MsgCABTmt"
  DFC_Msg2EBTmt/1 -> BMS_DSMR_FaultLvlCalc/161(DFC_Msg2EBTmt)  "DFC_Msg2EBTmt"
  DFC_Msg0B5Tmt/1 -> BMS_DSMR_FaultLvlCalc/163(DFC_Msg0B5Tmt)  "DFC_Msg0B5Tmt"
  DFC_ObcTmt/1 -> BMS_DSMR_FaultLvlCalc/164(DFC_ObcTmt)  "DFC_ObcTmt"
  DFC_VcuTmt/1 -> BMS_DSMR_FaultLvlCalc/165(DFC_VcuTmt)  "DFC_VcuTmt"
  DFC_Msg130Tmt/1 -> BMS_DSMR_FaultLvlCalc/159(DFC_Msg130Tmt)  "DFC_Msg130Tmt"
  DFC_Msg2E1Tmt/1 -> BMS_DSMR_FaultLvlCalc/160(DFC_Msg2E1Tmt)  "DFC_Msg2E1Tmt"
  DFC_Msg2ADTmt/1 -> BMS_DSMR_FaultLvlCalc/168(DFC_Msg2ADTmt)  "DFC_Msg2ADTmt"
  DFC_Msg2BBTmt/1 -> BMS_DSMR_FaultLvlCalc/169(DFC_Msg2BBTmt)  "DFC_Msg2BBTmt"
  DFC_Msg2A7Tmt/1 -> BMS_DSMR_FaultLvlCalc/166(DFC_Msg2A7Tmt)  "DFC_Msg2A7Tmt"
  DFC_Msg2A5Tmt/1 -> BMS_DSMR_FaultLvlCalc/167(DFC_Msg2A5Tmt)  "DFC_Msg2A5Tmt"
  DFC_Msg3AATmt/1 -> BMS_DSMR_FaultLvlCalc/171(DFC_Msg3AATmt)  "DFC_Msg3AATmt"
  DFC_Msg2DFTmt/1 -> BMS_DSMR_FaultLvlCalc/170(DFC_Msg2DFTmt)  "DFC_Msg2DFTmt"
  DFC_Msg050Tmt/1 -> BMS_DSMR_FaultLvlCalc/172(DFC_Msg050Tmt)  "DFC_Msg050Tmt"
  DFC_Msg2F1Tmt/1 -> BMS_DSMR_FaultLvlCalc/173(DFC_Msg2F1Tmt)  "DFC_Msg2F1Tmt"
  DFC_Msg37FTmt/1 -> BMS_DSMR_FaultLvlCalc/175(DFC_Msg37FTmt)  "DFC_Msg37FTmt"
  DFC_Msg195Tmt/1 -> BMS_DSMR_FaultLvlCalc/174(DFC_Msg195Tmt)  "DFC_Msg195Tmt"
  DFC_Msg17DTmt/1 -> BMS_DSMR_FaultLvlCalc/177(DFC_Msg17DTmt)  "DFC_Msg17DTmt"
  DFC_Msg28CTmt/1 -> BMS_DSMR_FaultLvlCalc/176(DFC_Msg28CTmt)  "DFC_Msg28CTmt"
  DFC_HwCurrElecSCP/1 -> BMS_DSMR_FaultLvlCalc/179(DFC_HwCurrElecSCP)  "DFC_HwCurrElecSCP"
  DFC_HwCurrElecSCG/1 -> BMS_DSMR_FaultLvlCalc/178(DFC_HwCurrElecSCG)  "DFC_HwCurrElecSCG"
  DFC_CABErr/1 -> BMS_DSMR_FaultLvlCalc/180(DFC_CABErr)  "DFC_CABErr"
  DFC_BattCurrMismatchErr/1 -> BMS_DSMR_FaultLvlCalc/181(DFC_BattCurrMismatchErr)  "DFC_BattCurrMismatchErr"
  GaCFM_AFEAdcRelatedErr_flg/1 -> BMS_DSMR_FaultLvlCalc/188(GaCFM_AFEAdcRelatedErr_flg)  "GaCFM_AFEAdcRelatedErr_flg"
  GaCFM_AFEGpioLineOpen_flg/1 -> BMS_DSMR_FaultLvlCalc/187(GaCFM_AFEGpioLineOpen_flg)  "GaCFM_AFEGpioLineOpen_flg"
  GaCFM_AFEDiagModeExitErr_flg/1 -> BMS_DSMR_FaultLvlCalc/189(GaCFM_AFEDiagModeExitErr_flg)  "GaCFM_AFEDiagModeExitErr_flg"
  GaCFM_AFECellVoltLineOpen_flg/1 -> BMS_DSMR_FaultLvlCalc/186(GaCFM_AFECellVoltLineOpen_flg)  "GaCFM_AFECellVoltLineOpen_flg"
  GaCFM_AFEOtherErr_flg/1 -> BMS_DSMR_FaultLvlCalc/190(GaCFM_AFEOtherErr_flg)  "GaCFM_AFEOtherErr_flg"
  GaCFM_AFESampleErr_flg/1 -> BMS_DSMR_FaultLvlCalc/185(GaCFM_AFESampleErr_flg)  "GaCFM_AFESampleErr_flg"
  GaCFM_AFECellTempUpdErr_flg/1 -> BMS_DSMR_FaultLvlCalc/184(GaCFM_AFECellTempUpdErr_flg)  "GaCFM_AFECellTempUpdErr_flg"
  GaCFM_AFECellVoltUpdErr_flg/1 -> BMS_DSMR_FaultLvlCalc/183(GaCFM_AFECellVoltUpdErr_flg)  "GaCFM_AFECellVoltUpdErr_flg"
  GaCFM_AFEComLost_flg/1 -> BMS_DSMR_FaultLvlCalc/182(GaCFM_AFEComLost_flg)  "GaCFM_AFEComLost_flg"
  DFC_AcDischgFobd/1 -> BMS_DSMR_FaultLvlCalc/191(DFC_AcDischgFobd)  "DFC_AcDischgFobd"
  DFC_BalCirOpenFlt/1 -> BMS_DSMR_FaultLvlCalc/192(DFC_BalCirOpenFlt)  "DFC_BalCirOpenFlt"
  DFC_BalCirShortFlt/1 -> BMS_DSMR_FaultLvlCalc/193(DFC_BalCirShortFlt)  "DFC_BalCirShortFlt"
  DFC_BalTempHighFlt/1 -> BMS_DSMR_FaultLvlCalc/194(DFC_BalTempHighFlt)  "DFC_BalTempHighFlt"
  DFC_HVSmplComFlt/1 -> BMS_DSMR_FaultLvlCalc/195(DFC_HVSmplComFlt)  "DFC_HVSmplComFlt"
  DFC_HVSmplSigErr/1 -> BMS_DSMR_FaultLvlCalc/196(DFC_HVSmplSigErr)  "DFC_HVSmplSigErr"
  DFC_HVSmplSplyFlt/1 -> BMS_DSMR_FaultLvlCalc/197(DFC_HVSmplSplyFlt)  "DFC_HVSmplSplyFlt"
  DFC_CABVoltOutOfRng/1 -> BMS_DSMR_FaultLvlCalc/198(DFC_CABVoltOutOfRng)  "DFC_CABVoltOutOfRng"
  DFC_CABDevFlt/1 -> BMS_DSMR_FaultLvlCalc/199(DFC_CABDevFlt)  "DFC_CABDevFlt"
  DFC_BMSSplyPwrAbnToLem/1 -> BMS_DSMR_FaultLvlCalc/200(DFC_BMSSplyPwrAbnToLem)  "DFC_BMSSplyPwrAbnToLem"
  DFC_BMSSplyPwrAbnToCAB/1 -> BMS_DSMR_FaultLvlCalc/201(DFC_BMSSplyPwrAbnToCAB)  "DFC_BMSSplyPwrAbnToCAB"
  DFC_NVMReadError/1 -> BMS_DSMR_FaultLvlCalc/202(DFC_NVMReadError)  "DFC_NVMReadError"
  DFC_KL30Shutdown/1 -> BMS_DSMR_FaultLvlCalc/203(DFC_KL30Shutdown)  "DFC_KL30Shutdown"
  DFC_MCUResetFlt/1 -> BMS_DSMR_FaultLvlCalc/204(DFC_MCUResetFlt)  "DFC_MCUResetFlt"
  DFC_BattSohChk/1 -> BMS_DSMR_FaultLvlCalc/205(DFC_BattSohChk)  "DFC_BattSohChk"
  DFC_CalCANBusOff/1 -> BMS_DSMR_FaultLvlCalc/206(DFC_CalCANBusOff)  "DFC_CalCANBusOff"
  DFC_ThmRnwyWarn/1 -> BMS_DSMR_FaultLvlCalc/207(DFC_ThmRnwyWarn)  "DFC_ThmRnwyWarn"
  DFC_PchgOvrCurrFlt/1 -> BMS_DSMR_FaultLvlCalc/208(DFC_PchgOvrCurrFlt)  "DFC_PchgOvrCurrFlt"
  DFC_SBCSplyPwrOvrVolt/1 -> BMS_DSMR_FaultLvlCalc/209(DFC_SBCSplyPwrOvrVolt)  "DFC_SBCSplyPwrOvrVolt"
  DFC_SBCSplyPwrUnderVolt/1 -> BMS_DSMR_FaultLvlCalc/210(DFC_SBCSplyPwrUnderVolt)  "DFC_SBCSplyPwrUnderVolt"
  DFC_SBCSplyPwrOvrCurr/1 -> BMS_DSMR_FaultLvlCalc/211(DFC_SBCSplyPwrOvrCurr)  "DFC_SBCSplyPwrOvrCurr"
  DFC_CrashChkHwFrqAbnorm/1 -> BMS_DSMR_FaultLvlCalc/212(DFC_CrashChkHwFrqAbnorm)  "DFC_CrashChkHwFrqAbnorm"
  DFC_CrashChkHwDutyAbnorm/1 -> BMS_DSMR_FaultLvlCalc/213(DFC_CrashChkHwDutyAbnorm)  "DFC_CrashChkHwDutyAbnorm"
  DFC_AFETempHighFlt/1 -> BMS_DSMR_FaultLvlCalc/214(DFC_AFETempHighFlt)  "DFC_AFETempHighFlt"
  DFC_PreHeatPtcErr/1 -> BMS_DSMR_FaultLvlCalc/232(DFC_PreHeatPtcErr)  "DFC_PreHeatPtcErr"
  DFC_PreHeatObcStatusErr/1 -> BMS_DSMR_FaultLvlCalc/231(DFC_PreHeatObcStatusErr)  "DFC_PreHeatObcStatusErr"
  DFC_PreHeatVcuReqTmt/1 -> BMS_DSMR_FaultLvlCalc/230(DFC_PreHeatVcuReqTmt)  "DFC_PreHeatVcuReqTmt"
  DFC_PreHeatErr/1 -> BMS_DSMR_FaultLvlCalc/229(DFC_PreHeatErr)  "DFC_PreHeatErr"
  DFC_AFESplyFlt/1 -> BMS_DSMR_FaultLvlCalc/228(DFC_AFESplyFlt)  "DFC_AFESplyFlt"
  DFC_AFEResetFlt/1 -> BMS_DSMR_FaultLvlCalc/227(DFC_AFEResetFlt)  "DFC_AFEResetFlt"
  DFC_EVCCDevFlt/1 -> BMS_DSMR_FaultLvlCalc/215(DFC_EVCCDevFlt)  "DFC_EVCCDevFlt"
  DFC_EVCCSplyPwrFlt/1 -> BMS_DSMR_FaultLvlCalc/216(DFC_EVCCSplyPwrFlt)  "DFC_EVCCSplyPwrFlt"
  DFC_EVCCVehComFlt/1 -> BMS_DSMR_FaultLvlCalc/217(DFC_EVCCVehComFlt)  "DFC_EVCCVehComFlt"
  DFC_EVCCPileComFlt/1 -> BMS_DSMR_FaultLvlCalc/218(DFC_EVCCPileComFlt)  "DFC_EVCCPileComFlt"
  DFC_EVCCVehHwFlt/1 -> BMS_DSMR_FaultLvlCalc/219(DFC_EVCCVehHwFlt)  "DFC_EVCCVehHwFlt"
  DFC_EVCCPileHwFlt/1 -> BMS_DSMR_FaultLvlCalc/220(DFC_EVCCPileHwFlt)  "DFC_EVCCPileHwFlt"
  DFC_IsoS1SwStuckOpen/1 -> BMS_DSMR_FaultLvlCalc/221(DFC_IsoS1SwStuckOpen)  "DFC_IsoS1SwStuckOpen"
  DFC_IsoS1SwStuckClsd/1 -> BMS_DSMR_FaultLvlCalc/222(DFC_IsoS1SwStuckClsd)  "DFC_IsoS1SwStuckClsd"
  DFC_IsoS2SwStuckOpen/1 -> BMS_DSMR_FaultLvlCalc/223(DFC_IsoS2SwStuckOpen)  "DFC_IsoS2SwStuckOpen"
  DFC_IsoS2SwStuckClsd/1 -> BMS_DSMR_FaultLvlCalc/224(DFC_IsoS2SwStuckClsd)  "DFC_IsoS2SwStuckClsd"
  DFC_IsoS3SwStuckOpen/1 -> BMS_DSMR_FaultLvlCalc/225(DFC_IsoS3SwStuckOpen)  "DFC_IsoS3SwStuckOpen"
  DFC_IsoS3SwStuckClsd/1 -> BMS_DSMR_FaultLvlCalc/226(DFC_IsoS3SwStuckClsd)  "DFC_IsoS3SwStuckClsd"
  DFC_MPosRlyDrvScb/1 -> BMS_DSMR_FaultLvlCalc/233(DFC_MPosRlyDrvScb)  "DFC_MPosRlyDrvScb"
  DFC_MPosRlyDrvScg/1 -> BMS_DSMR_FaultLvlCalc/234(DFC_MPosRlyDrvScg)  "DFC_MPosRlyDrvScg"
  DFC_MPosRlyDrvOL/1 -> BMS_DSMR_FaultLvlCalc/235(DFC_MPosRlyDrvOL)  "DFC_MPosRlyDrvOL"
  DFC_MposRlyDrvOvrCurr/1 -> BMS_DSMR_FaultLvlCalc/236(DFC_MposRlyDrvOvrCurr)  "DFC_MposRlyDrvOvrCurr"
  DFC_MPosRlyDrvFault/1 -> BMS_DSMR_FaultLvlCalc/237(DFC_MPosRlyDrvFault)  "DFC_MPosRlyDrvFault"
  DFC_MNegRlyDrvScb/1 -> BMS_DSMR_FaultLvlCalc/238(DFC_MNegRlyDrvScb)  "DFC_MNegRlyDrvScb"
  DFC_MNegRlyDrvScg/1 -> BMS_DSMR_FaultLvlCalc/239(DFC_MNegRlyDrvScg)  "DFC_MNegRlyDrvScg"
  DFC_MNegRlyDrvOL/1 -> BMS_DSMR_FaultLvlCalc/240(DFC_MNegRlyDrvOL)  "DFC_MNegRlyDrvOL"
  DFC_MNegRlyDrvOvrCurr/1 -> BMS_DSMR_FaultLvlCalc/241(DFC_MNegRlyDrvOvrCurr)  "DFC_MNegRlyDrvOvrCurr"
  DFC_MNegRlyDrvFault/1 -> BMS_DSMR_FaultLvlCalc/242(DFC_MNegRlyDrvFault)  "DFC_MNegRlyDrvFault"
  DFC_DcPosRlyDrvScb/1 -> BMS_DSMR_FaultLvlCalc/243(DFC_DcPosRlyDrvScb)  "DFC_DcPosRlyDrvScb"
  DFC_DcPosRlyDrvScg/1 -> BMS_DSMR_FaultLvlCalc/244(DFC_DcPosRlyDrvScg)  "DFC_DcPosRlyDrvScg"
  DFC_DcPosRlyDrvOL/1 -> BMS_DSMR_FaultLvlCalc/245(DFC_DcPosRlyDrvOL)  "DFC_DcPosRlyDrvOL"
  DFC_DChrgPosRlyDrvOvrCurr/1 -> BMS_DSMR_FaultLvlCalc/246(DFC_DChrgPosRlyDrvOvrCurr)  "DFC_DChrgPosRlyDrvOvrCurr"
  DFC_DcPosRlyDrvFault/1 -> BMS_DSMR_FaultLvlCalc/247(DFC_DcPosRlyDrvFault)  "DFC_DcPosRlyDrvFault"
  DFC_DcNegRlyDrvScb/1 -> BMS_DSMR_FaultLvlCalc/248(DFC_DcNegRlyDrvScb)  "DFC_DcNegRlyDrvScb"
  DFC_DcNegRlyDrvScg/1 -> BMS_DSMR_FaultLvlCalc/249(DFC_DcNegRlyDrvScg)  "DFC_DcNegRlyDrvScg"
  DFC_DcNegRlyDrvOL/1 -> BMS_DSMR_FaultLvlCalc/250(DFC_DcNegRlyDrvOL)  "DFC_DcNegRlyDrvOL"
  DFC_DChrgNegRlyDrvOvrCurr/1 -> BMS_DSMR_FaultLvlCalc/251(DFC_DChrgNegRlyDrvOvrCurr)  "DFC_DChrgNegRlyDrvOvrCurr"
  DFC_DcNegRlyDrvFault/1 -> BMS_DSMR_FaultLvlCalc/252(DFC_DcNegRlyDrvFault)  "DFC_DcNegRlyDrvFault"
  DFC_PreRlyDrvScb/1 -> BMS_DSMR_FaultLvlCalc/253(DFC_PreRlyDrvScb)  "DFC_PreRlyDrvScb"
  DFC_PreRlyDrvScg/1 -> BMS_DSMR_FaultLvlCalc/254(DFC_PreRlyDrvScg)  "DFC_PreRlyDrvScg"
  DFC_PreRlyDrvOL/1 -> BMS_DSMR_FaultLvlCalc/255(DFC_PreRlyDrvOL)  "DFC_PreRlyDrvOL"
  DFC_PrRlyDrvOvrCurr/1 -> BMS_DSMR_FaultLvlCalc/256(DFC_PrRlyDrvOvrCurr)  "DFC_PrRlyDrvOvrCurr"
  DFC_CellTAlrmMax/1 -> BMS_DSMR_FaultLvlCalc/257(DFC_CellTAlrmMax)  "DFC_CellTAlrmMax"
  DFC_CellTFaultMax/1 -> BMS_DSMR_FaultLvlCalc/258(DFC_CellTFaultMax)  "DFC_CellTFaultMax"
  DFC_CellTAlrmMin/1 -> BMS_DSMR_FaultLvlCalc/259(DFC_CellTAlrmMin)  "DFC_CellTAlrmMin"
  DFC_CellTFaultMin/1 -> BMS_DSMR_FaultLvlCalc/260(DFC_CellTFaultMin)  "DFC_CellTFaultMin"
  DFC_CellTempVldMin/1 -> BMS_DSMR_FaultLvlCalc/261(DFC_CellTempVldMin)  "DFC_CellTempVldMin"
  DFC_CellTCnstMax/1 -> BMS_DSMR_FaultLvlCalc/262(DFC_CellTCnstMax)  "DFC_CellTCnstMax"
  DFC_CellTGradtMax/1 -> BMS_DSMR_FaultLvlCalc/263(DFC_CellTGradtMax)  "DFC_CellTGradtMax"
  DFC_CellTWarnMax/1 -> BMS_DSMR_FaultLvlCalc/264(DFC_CellTWarnMax)  "DFC_CellTWarnMax"
  DFC_CellTWarnMin/1 -> BMS_DSMR_FaultLvlCalc/265(DFC_CellTWarnMin)  "DFC_CellTWarnMin"
  DFC_CellTempVldMax/1 -> BMS_DSMR_FaultLvlCalc/266(DFC_CellTempVldMax)  "DFC_CellTempVldMax"
  DFC_CellTHopMax/1 -> BMS_DSMR_FaultLvlCalc/267(DFC_CellTHopMax)  "DFC_CellTHopMax"
  DFC_TwoCurrSnsrFlt/1 -> BMS_DSMR_FaultLvlCalc/268(DFC_TwoCurrSnsrFlt)  "DFC_TwoCurrSnsrFlt"
  DFC_ThmRnwyAlarm/1 -> BMS_DSMR_FaultLvlCalc/269(DFC_ThmRnwyAlarm)  "DFC_ThmRnwyAlarm"
  DFC_ChkSumMsg2A5Err/1 -> BMS_DSMR_FaultLvlCalc/270(DFC_ChkSumMsg2A5Err)  "DFC_ChkSumMsg2A5Err"
  DFC_ChkSumMsg2A7Err/1 -> BMS_DSMR_FaultLvlCalc/271(DFC_ChkSumMsg2A7Err)  "DFC_ChkSumMsg2A7Err"
  DFC_DchrgIsoChkLv1/1 -> BMS_DSMR_FaultLvlCalc/272(DFC_DchrgIsoChkLv1)  "DFC_DchrgIsoChkLv1"
  DFC_DchrgIsoChkLv2/1 -> BMS_DSMR_FaultLvlCalc/273(DFC_DchrgIsoChkLv2)  "DFC_DchrgIsoChkLv2"
  DFC_HVOffIsoChkLv1/1 -> BMS_DSMR_FaultLvlCalc/274(DFC_HVOffIsoChkLv1)  "DFC_HVOffIsoChkLv1"
  DFC_HVOffIsoChkLv2/1 -> BMS_DSMR_FaultLvlCalc/275(DFC_HVOffIsoChkLv2)  "DFC_HVOffIsoChkLv2"
  DFC_PackCrntSaf/1 -> BMS_DSMR_FaultLvlCalc/276(DFC_PackCrntSaf)  "DFC_PackCrntSaf"
